FUNCTION "GESTIONE_ES" : VOID
TITLE =
{ S7_language := '9(1) Inglese (Stati Uniti)  11.01.2022  09:45:15' }
VERSION : 0.1


VAR_TEMP
  RETVAL : INT ;
  SetPointCamera_1 : REAL ;	//43FLA02 (camera riscaldo 1)
  SetPointCamera_2 : REAL ;	//44FLA02 (camera riscaldo 2)
  SetPointCamera_3 : REAL ;	//51FLA02 (camera riscaldo 3)
  SetPointCamera_4 : REAL ;	//52FLA02 (camera riscaldo 4)
  SetPointForno : REAL ;	//Forno
END_VAR
BEGIN
NETWORK
TITLE =**************************************

NETWORK
TITLE =Abilita Gestione Risparmio Energetico
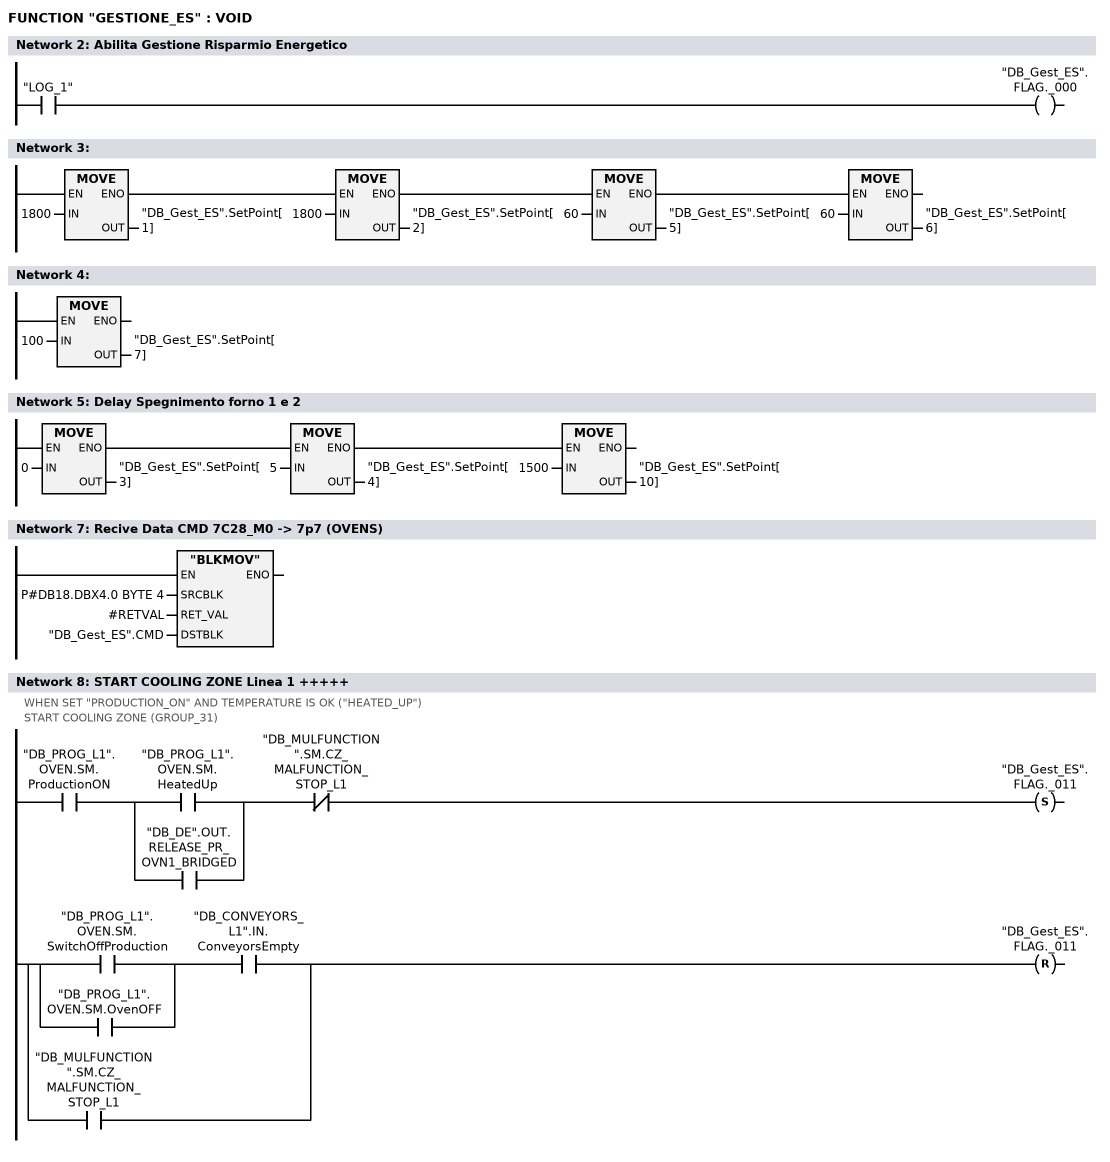
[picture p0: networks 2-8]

      U     "LOG_1";
      =     "DB_Gest_ES".FLAG._000;
NETWORK
TITLE =

      U(    ;
      U(    ;
      U(    ;
      L     1800;
      T     "DB_Gest_ES".SetPoint[1];
      SET   ;
      SAVE  ;
      CLR   ;
      U     BIE;
      )     ;
      SPBNB _001;
      L     1800;
      T     "DB_Gest_ES".SetPoint[2];
      SET   ;
      SAVE  ;
      CLR   ;
_001: U     BIE;
      )     ;
      SPBNB _002;
      L     60;
      T     "DB_Gest_ES".SetPoint[5];
      SET   ;
      SAVE  ;
      CLR   ;
_002: U     BIE;
      )     ;
      SPBNB _003;
      L     60;
      T     "DB_Gest_ES".SetPoint[6];
_003: NOP   0;
NETWORK
TITLE =

      L     100;
      T     "DB_Gest_ES".SetPoint[7];
      NOP   0;
NETWORK
TITLE =Delay Spegnimento forno 1 e 2

      U(    ;
      U(    ;
      L     0;
      T     "DB_Gest_ES".SetPoint[3];
      SET   ;
      SAVE  ;
      CLR   ;
      U     BIE;
      )     ;
      SPBNB _004;
      L     5;
      T     "DB_Gest_ES".SetPoint[4];
      SET   ;
      SAVE  ;
      CLR   ;
_004: U     BIE;
      )     ;
      SPBNB _005;
      L     1500;
      T     "DB_Gest_ES".SetPoint[10];
_005: NOP   0;
NETWORK
TITLE =**************************************

NETWORK
TITLE =Recive Data CMD 7C28_M0 -> 7p7 (OVENS)

      CALL "BLKMOV" (
           SRCBLK                   := P#DB18.DBX4.0 BYTE 4,
           RET_VAL                  := #RETVAL,
           DSTBLK                   := "DB_Gest_ES".CMD);
      NOP   0;
NETWORK
TITLE =START COOLING ZONE Linea 1 +++++
//WHEN SET "PRODUCTION_ON" AND TEMPERATURE IS OK ("HEATED_UP")
//START COOLING ZONE (GROUP_31)
      U     "DB_PROG_L1".OVEN.SM.ProductionON;
      U(    ;
      O     "DB_PROG_L1".OVEN.SM.HeatedUp;
      O     "DB_DE".OUT.RELEASE_PR_OVN1_BRIDGED;
      )     ;
      UN    "DB_MULFUNCTION".SM.CZ_MALFUNCTION_STOP_L1;
      S     "DB_Gest_ES".FLAG._011;
      U(    ;
      U(    ;
      O     "DB_PROG_L1".OVEN.SM.SwitchOffProduction;
      O     "DB_PROG_L1".OVEN.SM.OvenOFF;
      )     ;
      U     "DB_CONVEYORS_L1".IN.ConveyorsEmpty;
      O     "DB_MULFUNCTION".SM.CZ_MALFUNCTION_STOP_L1;
      )     ;
      R     "DB_Gest_ES".FLAG._011;
      NOP   0;
NETWORK
TITLE =Stop Raffreddamento Linea 1
//DB8.DBD38
      U     "DB_Gest_ES".FLAG._011;
      U     "DB_Gest_ES".FLAG._000;
      =     L     22.0;
      U     L     22.0;
      U(    ;
      U     "DB_Gest_ES".CMD.StopVentilazione_Zona1;
      UN    "DB_Gest_ES".FLAG._013;
      O     ;
      U     "DB_Gest_ES".Tmr.EN_Delay_01;
      UN    "DB_Gest_ES".Tmr.DN_Delay_01;
      )     ;
      S     "DB_Gest_ES".FLAG._001;
      U     L     22.0;
      UN    "DB_Gest_ES".CMD.StopVentilazione_Zona1;
      UN    "DB_Gest_ES".FLAG._013;
      S     "DB_Gest_ES".FLAG._013;
      U(    ;
      U     L     22.0;
      U     "DB_Gest_ES".CMD.VentilazioneRid_Zona1;
      =     "DB_Gest_ES".Tmr.EN_Delay_05;
      U     "DB_Gest_ES".Tmr.EN_Delay_05;
      )     ;
      U     "DB_Gest_ES".Tmr.DN_Delay_05;
      =     "DB_Gest_ES".FLAG._021;
NETWORK
TITLE =AUX Start Raff. Linea 1
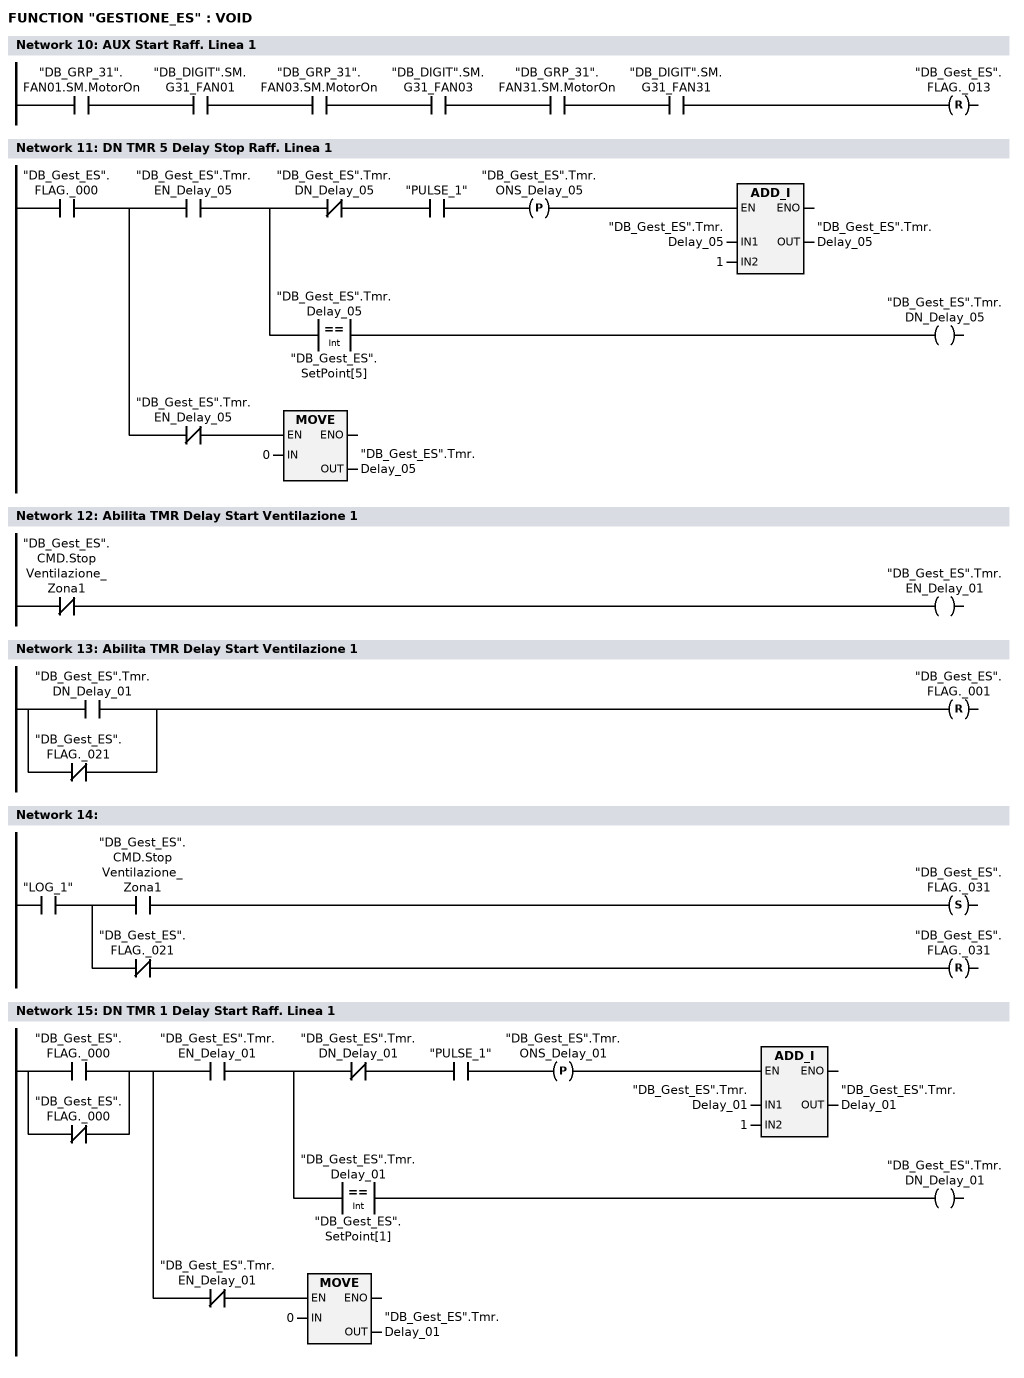
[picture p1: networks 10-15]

      U     "DB_GRP_31".FAN01.SM.MotorOn;
      U     "DB_DIGIT".SM.G31_FAN01;
      U     "DB_GRP_31".FAN03.SM.MotorOn;
      U     "DB_DIGIT".SM.G31_FAN03;
      U     "DB_GRP_31".FAN31.SM.MotorOn;
      U     "DB_DIGIT".SM.G31_FAN31;
      R     "DB_Gest_ES".FLAG._013;
NETWORK
TITLE =DN TMR 5 Delay Stop Raff. Linea 1

      U     "DB_Gest_ES".FLAG._000;
      =     L     22.0;
      U     L     22.0;
      U     "DB_Gest_ES".Tmr.EN_Delay_05;
      =     L     22.1;
      U     L     22.1;
      UN    "DB_Gest_ES".Tmr.DN_Delay_05;
      U     "PULSE_1";
      FP    "DB_Gest_ES".Tmr.ONS_Delay_05;
      SPBNB _006;
      L     "DB_Gest_ES".Tmr.Delay_05;
      L     1;
      +I    ;
      T     "DB_Gest_ES".Tmr.Delay_05;
_006: NOP   0;
      U     L     22.1;
      U(    ;
      L     "DB_Gest_ES".Tmr.Delay_05;
      L     "DB_Gest_ES".SetPoint[5];
      ==I   ;
      )     ;
      =     "DB_Gest_ES".Tmr.DN_Delay_05;
      U     L     22.0;
      UN    "DB_Gest_ES".Tmr.EN_Delay_05;
      SPBNB _007;
      L     0;
      T     "DB_Gest_ES".Tmr.Delay_05;
_007: NOP   0;
NETWORK
TITLE =Abilita TMR Delay Start Ventilazione 1

      UN    "DB_Gest_ES".CMD.StopVentilazione_Zona1;
      =     "DB_Gest_ES".Tmr.EN_Delay_01;
NETWORK
TITLE =Abilita TMR Delay Start Ventilazione 1

      O     "DB_Gest_ES".Tmr.DN_Delay_01;
      ON    "DB_Gest_ES".FLAG._021;
      R     "DB_Gest_ES".FLAG._001;
NETWORK
TITLE =

      U     "LOG_1";
      =     L     22.0;
      U     L     22.0;
      U     "DB_Gest_ES".CMD.StopVentilazione_Zona1;
      S     "DB_Gest_ES".FLAG._031;
      U     L     22.0;
      UN    "DB_Gest_ES".FLAG._021;
      R     "DB_Gest_ES".FLAG._031;
NETWORK
TITLE =DN TMR 1 Delay Start Raff. Linea 1

      O     "DB_Gest_ES".FLAG._000;
      ON    "DB_Gest_ES".FLAG._000;
      =     L     22.0;
      U     L     22.0;
      U     "DB_Gest_ES".Tmr.EN_Delay_01;
      =     L     22.1;
      U     L     22.1;
      UN    "DB_Gest_ES".Tmr.DN_Delay_01;
      U     "PULSE_1";
      FP    "DB_Gest_ES".Tmr.ONS_Delay_01;
      SPBNB _008;
      L     "DB_Gest_ES".Tmr.Delay_01;
      L     1;
      +I    ;
      T     "DB_Gest_ES".Tmr.Delay_01;
_008: NOP   0;
      U     L     22.1;
      U(    ;
      L     "DB_Gest_ES".Tmr.Delay_01;
      L     "DB_Gest_ES".SetPoint[1];
      ==I   ;
      )     ;
      =     "DB_Gest_ES".Tmr.DN_Delay_01;
      U     L     22.0;
      UN    "DB_Gest_ES".Tmr.EN_Delay_01;
      SPBNB _009;
      L     0;
      T     "DB_Gest_ES".Tmr.Delay_01;
_009: NOP   0;
NETWORK
TITLE =Stop Riscaldamento Linea 1

      U     "LOG_0";
      =     L     22.0;
      U(    ;
      U     L     22.0;
      U     "DB_Gest_ES".FLAG._000;
      U     "DB_CalendarioF1".CMD_OFF;
      U     "DB_CalendarioF1".Auto;
      UN    "DB_PROG_L1".OVEN.SM.SwitchOffProduction;
      U     "DB_Gest_ES".CMD.Stop_Riscarldo_Forno1;
      U     "DB_Gest_ES".CMD.AssenzaScoccheCabina;
      =     "DB_Gest_ES".Tmr.EN_Delay_03;
      U     "DB_Gest_ES".Tmr.EN_Delay_03;
      )     ;
      U     "DB_Gest_ES".Tmr.DN_Delay_03;
      S     "DB_Gest_ES".FLAG._003;
      R     "DB_CalendarioF1".CMD_OFF;
      U     L     22.0;
      U(    ;
      O     "DB_PROG_L1".OVEN.SM.SwitchOffProduction;
      O     "DB_PROG_L1".OVEN.SM.OvenOFF;
      O     "DB_PROG_L1".OVEN.CTRL.PreHeatingOn;
      O     "DB_PROG_L1".OVEN.CTRL.ProductionOn;
      )     ;
      R     "DB_Gest_ES".FLAG._003;
NETWORK
TITLE =
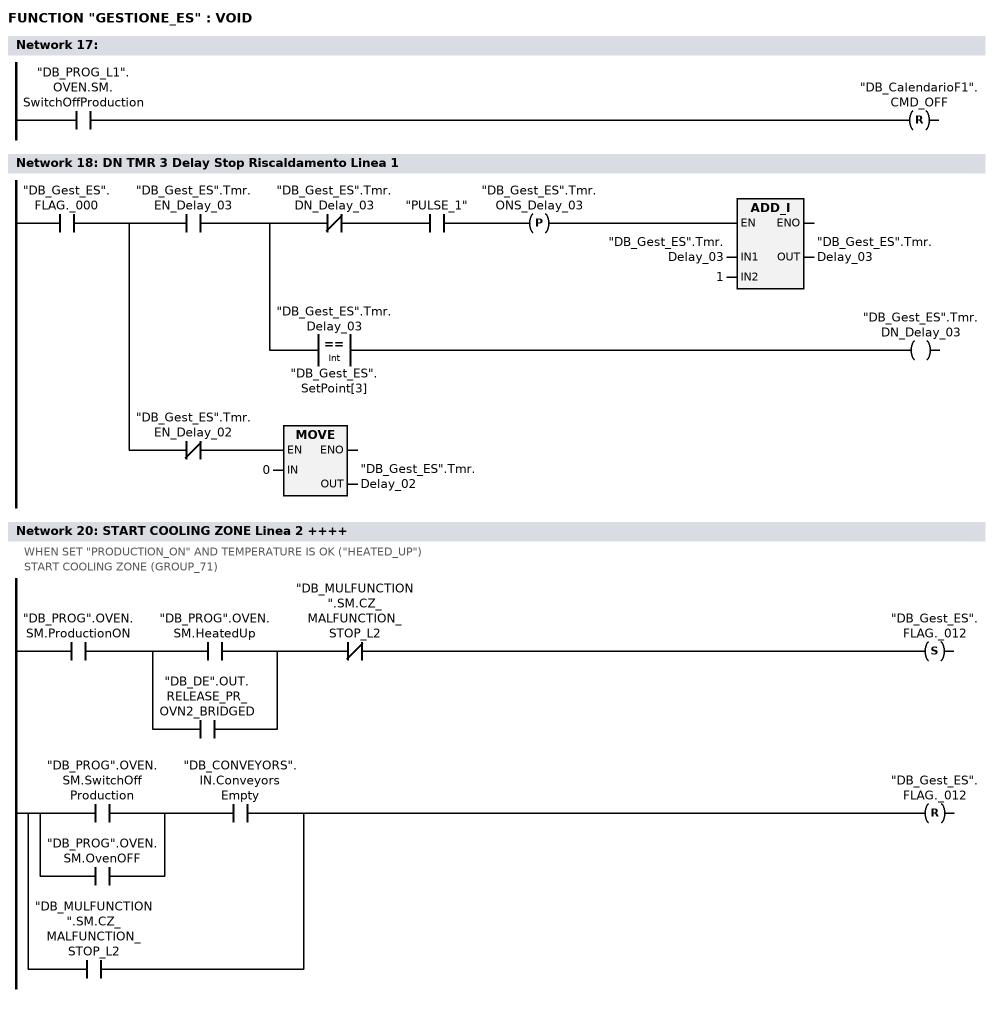
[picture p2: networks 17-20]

      U     "DB_PROG_L1".OVEN.SM.SwitchOffProduction;
      R     "DB_CalendarioF1".CMD_OFF;
NETWORK
TITLE =DN TMR 3 Delay Stop Riscaldamento Linea 1

      U     "DB_Gest_ES".FLAG._000;
      =     L     22.0;
      U     L     22.0;
      U     "DB_Gest_ES".Tmr.EN_Delay_03;
      =     L     22.1;
      U     L     22.1;
      UN    "DB_Gest_ES".Tmr.DN_Delay_03;
      U     "PULSE_1";
      FP    "DB_Gest_ES".Tmr.ONS_Delay_03;
      SPBNB _00a;
      L     "DB_Gest_ES".Tmr.Delay_03;
      L     1;
      +I    ;
      T     "DB_Gest_ES".Tmr.Delay_03;
_00a: NOP   0;
      U     L     22.1;
      U(    ;
      L     "DB_Gest_ES".Tmr.Delay_03;
      L     "DB_Gest_ES".SetPoint[3];
      ==I   ;
      )     ;
      =     "DB_Gest_ES".Tmr.DN_Delay_03;
      U     L     22.0;
      UN    "DB_Gest_ES".Tmr.EN_Delay_02;
      SPBNB _00b;
      L     0;
      T     "DB_Gest_ES".Tmr.Delay_02;
_00b: NOP   0;
NETWORK
TITLE =**************************************

NETWORK
TITLE =START COOLING ZONE Linea 2 ++++
//WHEN SET "PRODUCTION_ON" AND TEMPERATURE IS OK ("HEATED_UP")
//START COOLING ZONE (GROUP_71)
      U     "DB_PROG".OVEN.SM.ProductionON;
      U(    ;
      O     "DB_PROG".OVEN.SM.HeatedUp;
      O     "DB_DE".OUT.RELEASE_PR_OVN2_BRIDGED;
      )     ;
      UN    "DB_MULFUNCTION".SM.CZ_MALFUNCTION_STOP_L2;
      S     "DB_Gest_ES".FLAG._012;
      U(    ;
      U(    ;
      O     "DB_PROG".OVEN.SM.SwitchOffProduction;
      O     "DB_PROG".OVEN.SM.OvenOFF;
      )     ;
      U     "DB_CONVEYORS".IN.ConveyorsEmpty;
      O     "DB_MULFUNCTION".SM.CZ_MALFUNCTION_STOP_L2;
      )     ;
      R     "DB_Gest_ES".FLAG._012;
      NOP   0;
NETWORK
TITLE =Stop Raffreddamento Linea 2
//DB8.DBD38
      U     "DB_Gest_ES".FLAG._012;
      U     "DB_Gest_ES".FLAG._000;
      U     "LOG_0";
      =     L     22.0;
      U     L     22.0;
      U(    ;
      U     "DB_Gest_ES".CMD.StopVentilazione_Zona2;
      UN    "DB_Gest_ES".FLAG._014;
      O     ;
      U     "DB_Gest_ES".Tmr.EN_Delay_02;
      UN    "DB_Gest_ES".Tmr.DN_Delay_02;
      )     ;
      S     "DB_Gest_ES".FLAG._002;
      U     L     22.0;
      UN    "DB_Gest_ES".CMD.StopVentilazione_Zona2;
      UN    "DB_Gest_ES".FLAG._014;
      S     "DB_Gest_ES".FLAG._014;
      U(    ;
      U     L     22.0;
      U     "DB_Gest_ES".CMD.VentilazioneRid_Zona2;
      =     "DB_Gest_ES".Tmr.EN_Delay_06;
      U     "DB_Gest_ES".Tmr.EN_Delay_06;
      )     ;
      U     "DB_Gest_ES".Tmr.DN_Delay_06;
      =     "DB_Gest_ES".FLAG._022;
NETWORK
TITLE =AUX Start Raff. Linea 2
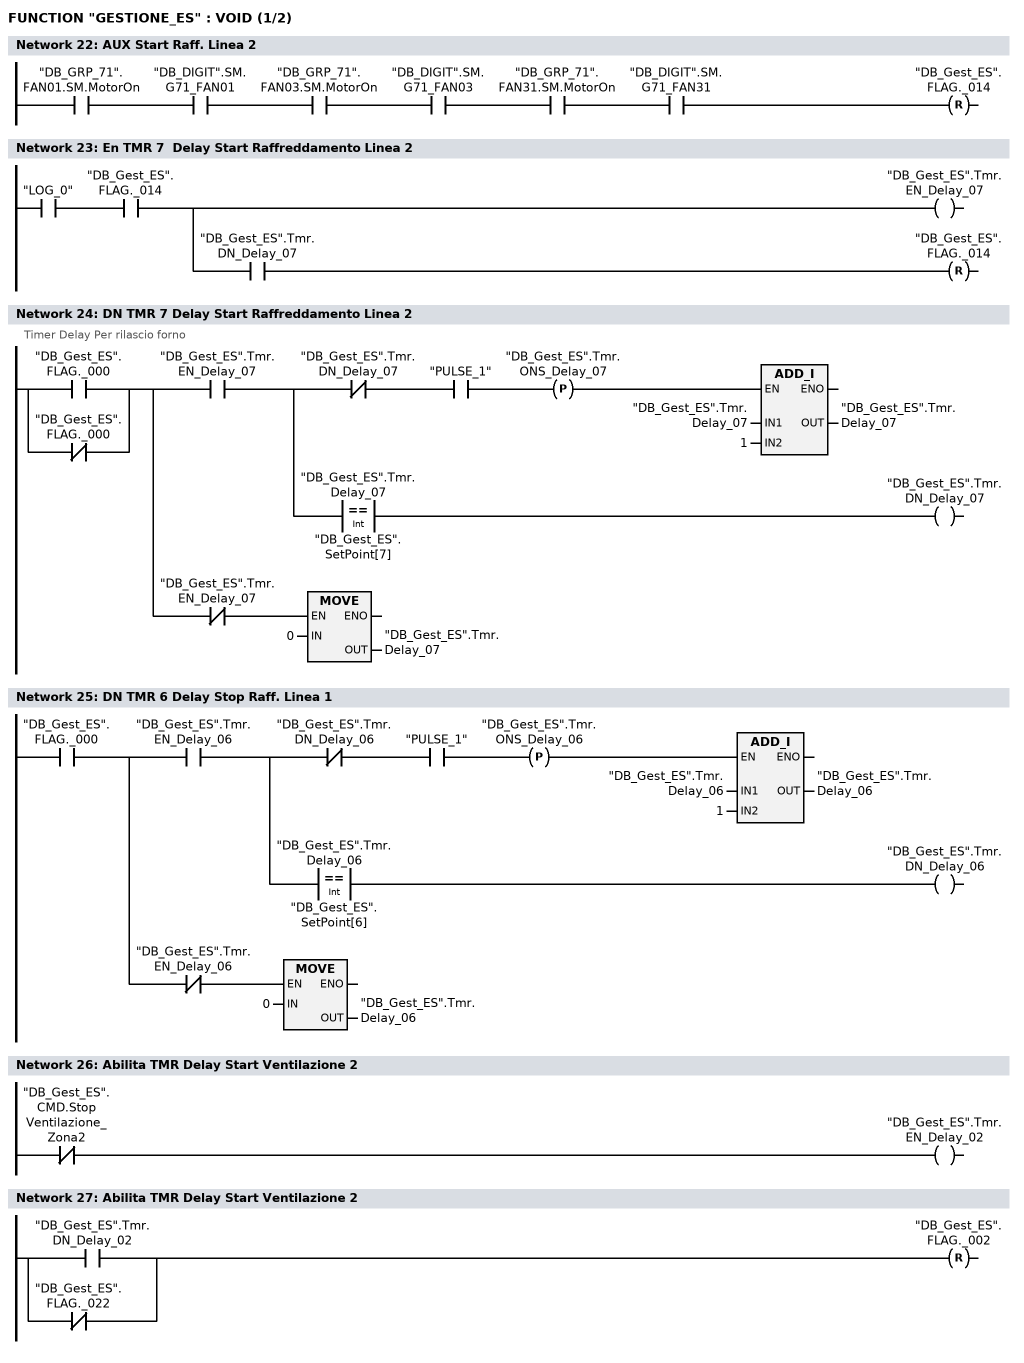
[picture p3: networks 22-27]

      U     "DB_GRP_71".FAN01.SM.MotorOn;
      U     "DB_DIGIT".SM.G71_FAN01;
      U     "DB_GRP_71".FAN03.SM.MotorOn;
      U     "DB_DIGIT".SM.G71_FAN03;
      U     "DB_GRP_71".FAN31.SM.MotorOn;
      U     "DB_DIGIT".SM.G71_FAN31;
      R     "DB_Gest_ES".FLAG._014;
NETWORK
TITLE =En TMR 7  Delay Start Raffreddamento Linea 2

      U     "LOG_0";
      U     "DB_Gest_ES".FLAG._014;
      =     L     22.0;
      U     L     22.0;
      BLD   102;
      =     "DB_Gest_ES".Tmr.EN_Delay_07;
      U     L     22.0;
      U     "DB_Gest_ES".Tmr.DN_Delay_07;
      R     "DB_Gest_ES".FLAG._014;
NETWORK
TITLE =DN TMR 7 Delay Start Raffreddamento Linea 2
//Timer Delay Per rilascio forno
      O     "DB_Gest_ES".FLAG._000;
      ON    "DB_Gest_ES".FLAG._000;
      =     L     22.0;
      U     L     22.0;
      U     "DB_Gest_ES".Tmr.EN_Delay_07;
      =     L     22.1;
      U     L     22.1;
      UN    "DB_Gest_ES".Tmr.DN_Delay_07;
      U     "PULSE_1";
      FP    "DB_Gest_ES".Tmr.ONS_Delay_07;
      SPBNB _00c;
      L     "DB_Gest_ES".Tmr.Delay_07;
      L     1;
      +I    ;
      T     "DB_Gest_ES".Tmr.Delay_07;
_00c: NOP   0;
      U     L     22.1;
      U(    ;
      L     "DB_Gest_ES".Tmr.Delay_07;
      L     "DB_Gest_ES".SetPoint[7];
      ==I   ;
      )     ;
      =     "DB_Gest_ES".Tmr.DN_Delay_07;
      U     L     22.0;
      UN    "DB_Gest_ES".Tmr.EN_Delay_07;
      SPBNB _00d;
      L     0;
      T     "DB_Gest_ES".Tmr.Delay_07;
_00d: NOP   0;
NETWORK
TITLE =DN TMR 6 Delay Stop Raff. Linea 1

      U     "DB_Gest_ES".FLAG._000;
      =     L     22.0;
      U     L     22.0;
      U     "DB_Gest_ES".Tmr.EN_Delay_06;
      =     L     22.1;
      U     L     22.1;
      UN    "DB_Gest_ES".Tmr.DN_Delay_06;
      U     "PULSE_1";
      FP    "DB_Gest_ES".Tmr.ONS_Delay_06;
      SPBNB _00e;
      L     "DB_Gest_ES".Tmr.Delay_06;
      L     1;
      +I    ;
      T     "DB_Gest_ES".Tmr.Delay_06;
_00e: NOP   0;
      U     L     22.1;
      U(    ;
      L     "DB_Gest_ES".Tmr.Delay_06;
      L     "DB_Gest_ES".SetPoint[6];
      ==I   ;
      )     ;
      =     "DB_Gest_ES".Tmr.DN_Delay_06;
      U     L     22.0;
      UN    "DB_Gest_ES".Tmr.EN_Delay_06;
      SPBNB _00f;
      L     0;
      T     "DB_Gest_ES".Tmr.Delay_06;
_00f: NOP   0;
NETWORK
TITLE =Abilita TMR Delay Start Ventilazione 2

      UN    "DB_Gest_ES".CMD.StopVentilazione_Zona2;
      =     "DB_Gest_ES".Tmr.EN_Delay_02;
NETWORK
TITLE =Abilita TMR Delay Start Ventilazione 2

      O     "DB_Gest_ES".Tmr.DN_Delay_02;
      ON    "DB_Gest_ES".FLAG._022;
      R     "DB_Gest_ES".FLAG._002;
NETWORK
TITLE =DN TMR 2 Delay Stop Riscaldamento Linea 2
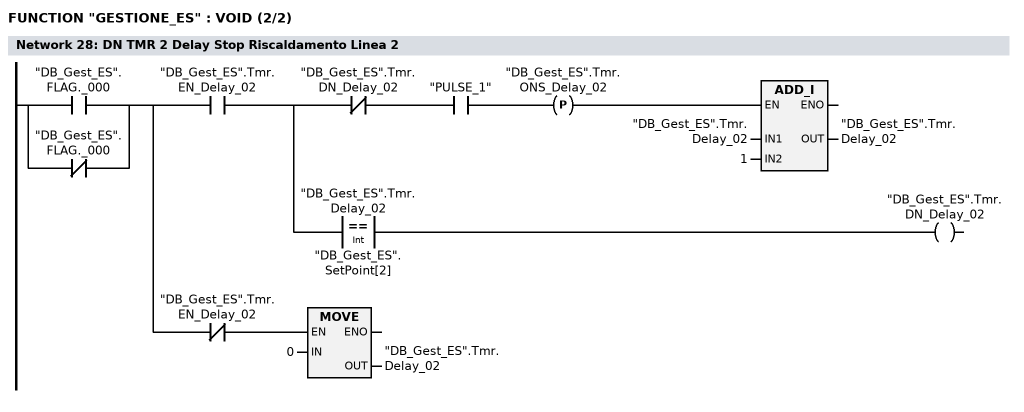
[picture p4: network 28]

      O     "DB_Gest_ES".FLAG._000;
      ON    "DB_Gest_ES".FLAG._000;
      =     L     22.0;
      U     L     22.0;
      U     "DB_Gest_ES".Tmr.EN_Delay_02;
      =     L     22.1;
      U     L     22.1;
      UN    "DB_Gest_ES".Tmr.DN_Delay_02;
      U     "PULSE_1";
      FP    "DB_Gest_ES".Tmr.ONS_Delay_02;
      SPBNB _010;
      L     "DB_Gest_ES".Tmr.Delay_02;
      L     1;
      +I    ;
      T     "DB_Gest_ES".Tmr.Delay_02;
_010: NOP   0;
      U     L     22.1;
      U(    ;
      L     "DB_Gest_ES".Tmr.Delay_02;
      L     "DB_Gest_ES".SetPoint[2];
      ==I   ;
      )     ;
      =     "DB_Gest_ES".Tmr.DN_Delay_02;
      U     L     22.0;
      UN    "DB_Gest_ES".Tmr.EN_Delay_02;
      SPBNB _011;
      L     0;
      T     "DB_Gest_ES".Tmr.Delay_02;
_011: NOP   0;
NETWORK
TITLE =Stop Riscaldamento Linea 2

      U     "LOG_1";
      =     L     22.0;
      U(    ;
      U     L     22.0;
      U     "DB_Gest_ES".FLAG._000;
      U     "DB_CalendarioF2".CMD_OFF;
      U     "DB_CalendarioF2".Auto;
      UN    "DB_PROG".OVEN.SM.SwitchOffProduction;
      U     "DB_Gest_ES".CMD.AssenzaScoccheCabina;
      =     "DB_Gest_ES".Tmr.EN_Delay_04;
      U     "DB_Gest_ES".Tmr.EN_Delay_04;
      )     ;
      U     "DB_Gest_ES".CMD.Stop_Riscarldo_Forno2;
      U     "DB_Gest_ES".Tmr.DN_Delay_04;
      U     "DB_Gest_ES".Tmr.DN_Delay_10;
      S     "DB_Gest_ES".FLAG._004;
      S     "DB_Gest_ES".FLAG._005;
      R     "DB_CalendarioF2".CMD_OFF;
      R     "DB_Gest_ES".FLAG._050;
      U     L     22.0;
      U(    ;
      U     "DB_PROG".OVEN.SM.SwitchOffProduction;
      UN    "DB_PROG".OVEN.SM.ProductionON;
      O     "DB_PROG".OVEN.SM.OvenOFF;
      O     "DB_PROG".OVEN.CTRL.PreHeatingOn;
      O     "DB_PROG".OVEN.CTRL.ProductionOn;
      )     ;
      R     "DB_Gest_ES".FLAG._004;
NETWORK
TITLE =RESET COMANDO OFF
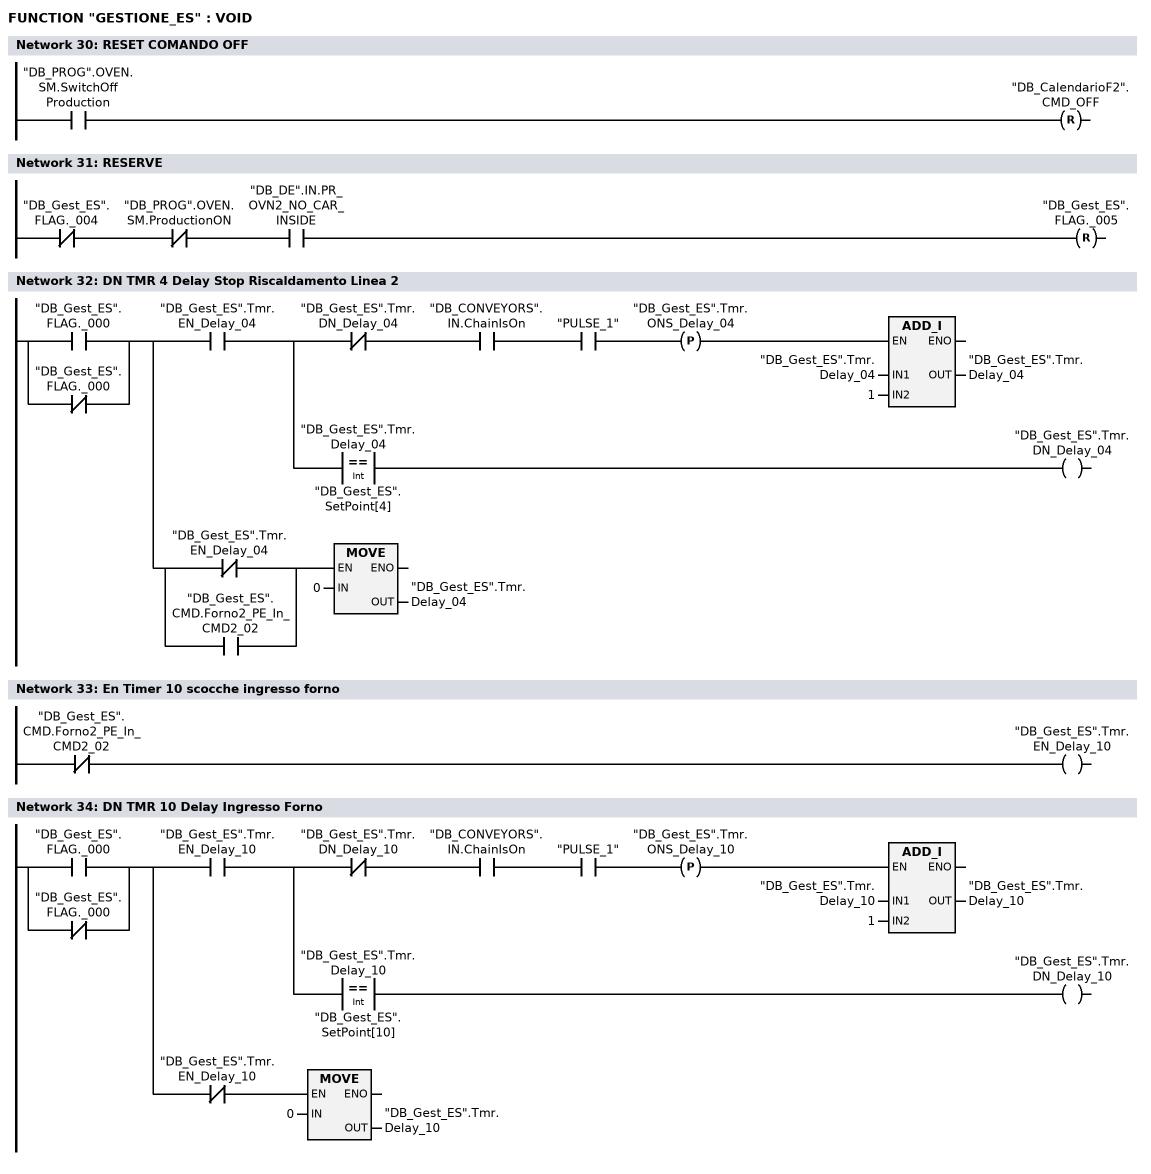
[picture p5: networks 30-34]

      U     "DB_PROG".OVEN.SM.SwitchOffProduction;
      R     "DB_CalendarioF2".CMD_OFF;
NETWORK
TITLE =RESERVE

      UN    "DB_Gest_ES".FLAG._004;
      UN    "DB_PROG".OVEN.SM.ProductionON;
      U     "DB_DE".IN.PR_OVN2_NO_CAR_INSIDE;
      R     "DB_Gest_ES".FLAG._005;
NETWORK
TITLE =DN TMR 4 Delay Stop Riscaldamento Linea 2

      O     "DB_Gest_ES".FLAG._000;
      ON    "DB_Gest_ES".FLAG._000;
      =     L     22.0;
      U     L     22.0;
      U     "DB_Gest_ES".Tmr.EN_Delay_04;
      =     L     22.1;
      U     L     22.1;
      UN    "DB_Gest_ES".Tmr.DN_Delay_04;
      U     "DB_CONVEYORS".IN.ChainIsOn;
      U     "PULSE_1";
      FP    "DB_Gest_ES".Tmr.ONS_Delay_04;
      SPBNB _012;
      L     "DB_Gest_ES".Tmr.Delay_04;
      L     1;
      +I    ;
      T     "DB_Gest_ES".Tmr.Delay_04;
_012: NOP   0;
      U     L     22.1;
      U(    ;
      L     "DB_Gest_ES".Tmr.Delay_04;
      L     "DB_Gest_ES".SetPoint[4];
      ==I   ;
      )     ;
      =     "DB_Gest_ES".Tmr.DN_Delay_04;
      U     L     22.0;
      U(    ;
      ON    "DB_Gest_ES".Tmr.EN_Delay_04;
      O     "DB_Gest_ES".CMD.Forno2_PE_In_CMD2_02;
      )     ;
      SPBNB _013;
      L     0;
      T     "DB_Gest_ES".Tmr.Delay_04;
_013: NOP   0;
NETWORK
TITLE =En Timer 10 scocche ingresso forno

      UN    "DB_Gest_ES".CMD.Forno2_PE_In_CMD2_02;
      =     "DB_Gest_ES".Tmr.EN_Delay_10;
NETWORK
TITLE =DN TMR 10 Delay Ingresso Forno

      O     "DB_Gest_ES".FLAG._000;
      ON    "DB_Gest_ES".FLAG._000;
      =     L     22.0;
      U     L     22.0;
      U     "DB_Gest_ES".Tmr.EN_Delay_10;
      =     L     22.1;
      U     L     22.1;
      UN    "DB_Gest_ES".Tmr.DN_Delay_10;
      U     "DB_CONVEYORS".IN.ChainIsOn;
      U     "PULSE_1";
      FP    "DB_Gest_ES".Tmr.ONS_Delay_10;
      SPBNB _014;
      L     "DB_Gest_ES".Tmr.Delay_10;
      L     1;
      +I    ;
      T     "DB_Gest_ES".Tmr.Delay_10;
_014: NOP   0;
      U     L     22.1;
      U(    ;
      L     "DB_Gest_ES".Tmr.Delay_10;
      L     "DB_Gest_ES".SetPoint[10];
      ==I   ;
      )     ;
      =     "DB_Gest_ES".Tmr.DN_Delay_10;
      U     L     22.0;
      UN    "DB_Gest_ES".Tmr.EN_Delay_10;
      SPBNB _015;
      L     0;
      T     "DB_Gest_ES".Tmr.Delay_10;
_015: NOP   0;
NETWORK
TITLE =**************************************

NETWORK
TITLE =######################################

NETWORK
TITLE =Send Data CMD 7P7 -> 7C28_M0

NETWORK
TITLE =######################################

NETWORK
TITLE =#CALENDARIO FORNO 1

NETWORK
TITLE =Set
//Anno
      L     DB3100.DBB    8;
      T     "DB_CalendarioF1".PLC.Year;
//Mese
      L     DB3100.DBB    9;
      T     "DB_CalendarioF1".PLC.Mon;
//Giorno
      L     DB3100.DBB   10;
      T     "DB_CalendarioF1".PLC.Day;


//Ore
      L     DB3100.DBB   11;
      BTI   ;
      T     "DB_CalendarioF1".PLC.Hour;
//Minuti
      L     DB3100.DBB   12;
      BTI   ;
      T     "DB_CalendarioF1".PLC.Min;



NETWORK
TITLE =Calcolo del giorno della settimana

      L     DB3100.DBB   15;
      UW    W#16#F;
      T     "DB_CalendarioF1".PLC.WeekDay;
NETWORK
TITLE =Richiamo FC Gestione calendario
//P#DB101.DBX 50.0 BYTE 4
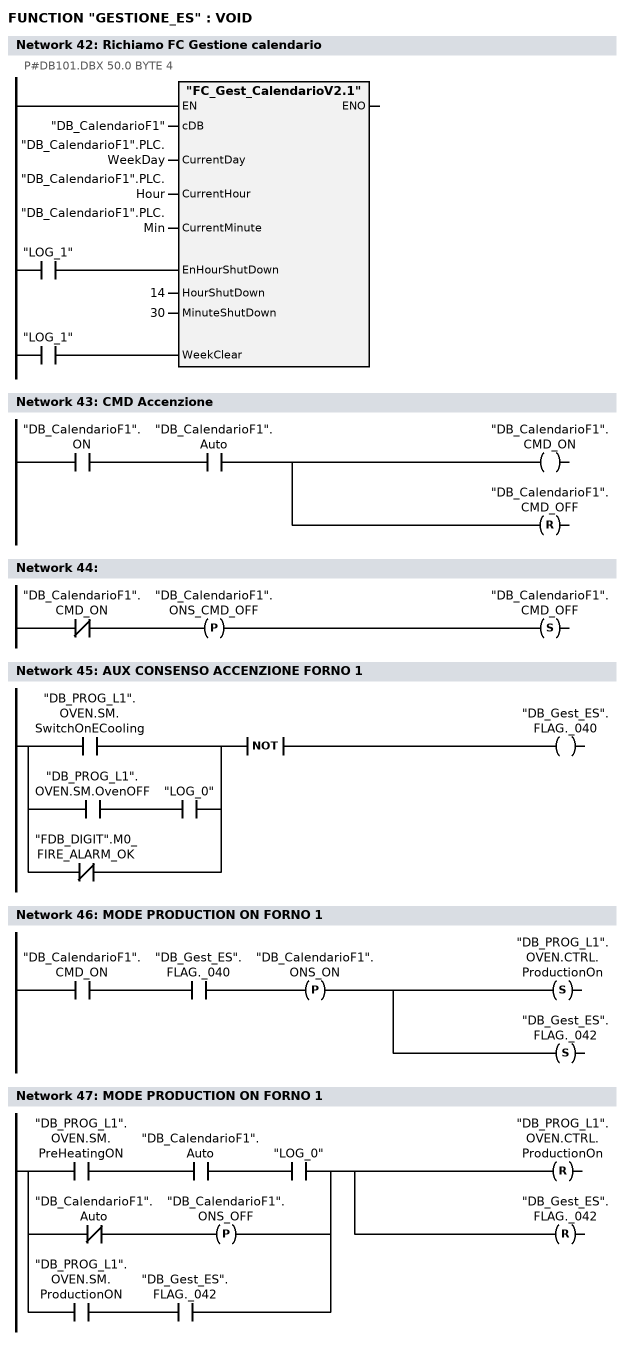
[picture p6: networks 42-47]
      U     "LOG_1";
      =     L     22.0;
      BLD   103;
      U     "LOG_1";
      =     L     22.1;
      BLD   103;
      CALL "FC_Gest_CalendarioV2.1" (
           cDB                      := "DB_CalendarioF1",
           CurrentDay               := "DB_CalendarioF1".PLC.WeekDay,
           CurrentHour              := "DB_CalendarioF1".PLC.Hour,
           CurrentMinute            := "DB_CalendarioF1".PLC.Min,
           EnHourShutDown           := L     22.0,
           HourShutDown             := 14,
           MinuteShutDown           := 30,
           WeekClear                := L     22.1);
      NOP   0;
NETWORK
TITLE =CMD Accenzione

      U     "DB_CalendarioF1".ON;
      U     "DB_CalendarioF1".Auto;
      =     "DB_CalendarioF1".CMD_ON;
      R     "DB_CalendarioF1".CMD_OFF;
NETWORK
TITLE =

      UN    "DB_CalendarioF1".CMD_ON;
      FP    "DB_CalendarioF1".ONS_CMD_OFF;
      S     "DB_CalendarioF1".CMD_OFF;
NETWORK
TITLE =AUX CONSENSO ACCENZIONE FORNO 1

      U(    ;
      O     "DB_PROG_L1".OVEN.SM.SwitchOnECooling;
      O     ;
      U     "DB_PROG_L1".OVEN.SM.OvenOFF;
      U     "LOG_0";
      ON    "FDB_DIGIT".M0_FIRE_ALARM_OK;
      )     ;
      NOT   ;
      =     "DB_Gest_ES".FLAG._040;
NETWORK
TITLE =MODE PRODUCTION ON FORNO 1

      U     "DB_CalendarioF1".CMD_ON;
      U     "DB_Gest_ES".FLAG._040;
      FP    "DB_CalendarioF1".ONS_ON;
      S     "DB_PROG_L1".OVEN.CTRL.ProductionOn;
      S     "DB_Gest_ES".FLAG._042;
NETWORK
TITLE =MODE PRODUCTION ON FORNO 1

      U     "DB_PROG_L1".OVEN.SM.PreHeatingON;
      U     "DB_CalendarioF1".Auto;
      U     "LOG_0";
      O(    ;
      UN    "DB_CalendarioF1".Auto;
      FP    "DB_CalendarioF1".ONS_OFF;
      )     ;
      O     ;
      U     "DB_PROG_L1".OVEN.SM.ProductionON;
      U     "DB_Gest_ES".FLAG._042;
      R     "DB_PROG_L1".OVEN.CTRL.ProductionOn;
      R     "DB_Gest_ES".FLAG._042;
NETWORK
TITLE =######################################

NETWORK
TITLE =#CALENDARIO FORNO 2

NETWORK
TITLE =Set
//Anno
      L     DB3100.DBB    8;
      T     "DB_CalendarioF2".PLC.Year;
//Mese
      L     DB3100.DBB    9;
      T     "DB_CalendarioF2".PLC.Mon;
//Giorno
      L     DB3100.DBB   10;
      T     "DB_CalendarioF2".PLC.Day;


//Ore
      L     DB3100.DBB   11;
      BTI   ;
      T     "DB_CalendarioF2".PLC.Hour;
//Minuti
      L     DB3100.DBB   12;
      BTI   ;
      T     "DB_CalendarioF2".PLC.Min;



NETWORK
TITLE =Calcolo del giorno della settimana

      L     DB3100.DBB   15;
      UW    W#16#F;
      T     "DB_CalendarioF2".PLC.WeekDay;
NETWORK
TITLE =Richiamo FC Gestione calendario
//P#DB101.DBX 50.0 BYTE 4
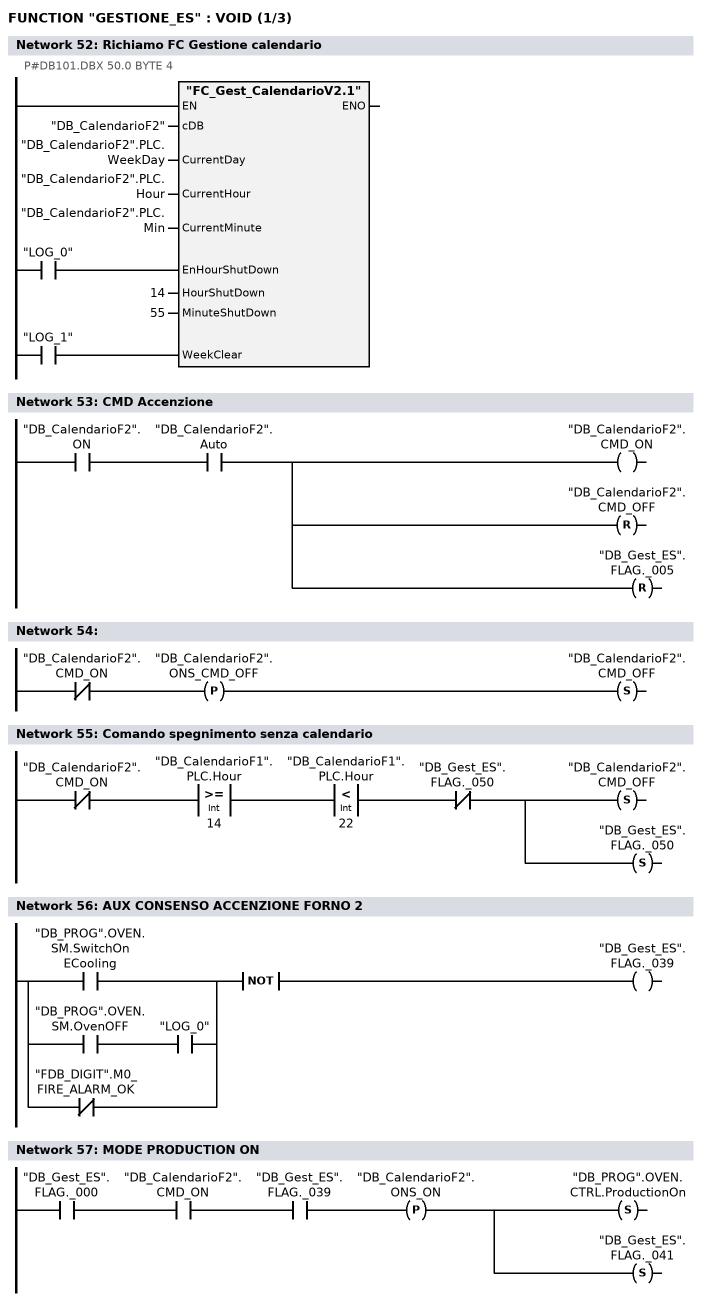
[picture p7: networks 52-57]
      U     "LOG_0";
      =     L     22.0;
      BLD   103;
      U     "LOG_1";
      =     L     22.1;
      BLD   103;
      CALL "FC_Gest_CalendarioV2.1" (
           cDB                      := "DB_CalendarioF2",
           CurrentDay               := "DB_CalendarioF2".PLC.WeekDay,
           CurrentHour              := "DB_CalendarioF2".PLC.Hour,
           CurrentMinute            := "DB_CalendarioF2".PLC.Min,
           EnHourShutDown           := L     22.0,
           HourShutDown             := 14,
           MinuteShutDown           := 55,
           WeekClear                := L     22.1);
      NOP   0;
NETWORK
TITLE =CMD Accenzione

      U     "DB_CalendarioF2".ON;
      U     "DB_CalendarioF2".Auto;
      =     "DB_CalendarioF2".CMD_ON;
      R     "DB_CalendarioF2".CMD_OFF;
      R     "DB_Gest_ES".FLAG._005;
NETWORK
TITLE =

      UN    "DB_CalendarioF2".CMD_ON;
      FP    "DB_CalendarioF2".ONS_CMD_OFF;
      S     "DB_CalendarioF2".CMD_OFF;
NETWORK
TITLE =Comando spegnimento senza calendario

      UN    "DB_CalendarioF2".CMD_ON;
      U(    ;
      L     "DB_CalendarioF1".PLC.Hour;
      L     14;
      >=I   ;
      )     ;
      U(    ;
      L     "DB_CalendarioF1".PLC.Hour;
      L     22;
      <I    ;
      )     ;
      UN    "DB_Gest_ES".FLAG._050;
      S     "DB_CalendarioF2".CMD_OFF;
      S     "DB_Gest_ES".FLAG._050;
NETWORK
TITLE =AUX CONSENSO ACCENZIONE FORNO 2

      U(    ;
      O     "DB_PROG".OVEN.SM.SwitchOnECooling;
      O     ;
      U     "DB_PROG".OVEN.SM.OvenOFF;
      U     "LOG_0";
      ON    "FDB_DIGIT".M0_FIRE_ALARM_OK;
      )     ;
      NOT   ;
      =     "DB_Gest_ES".FLAG._039;
NETWORK
TITLE =MODE PRODUCTION ON

      U     "DB_Gest_ES".FLAG._000;
      U     "DB_CalendarioF2".CMD_ON;
      U     "DB_Gest_ES".FLAG._039;
      FP    "DB_CalendarioF2".ONS_ON;
      S     "DB_PROG".OVEN.CTRL.ProductionOn;
      S     "DB_Gest_ES".FLAG._041;
NETWORK
TITLE =MODE PRODUCTION ON
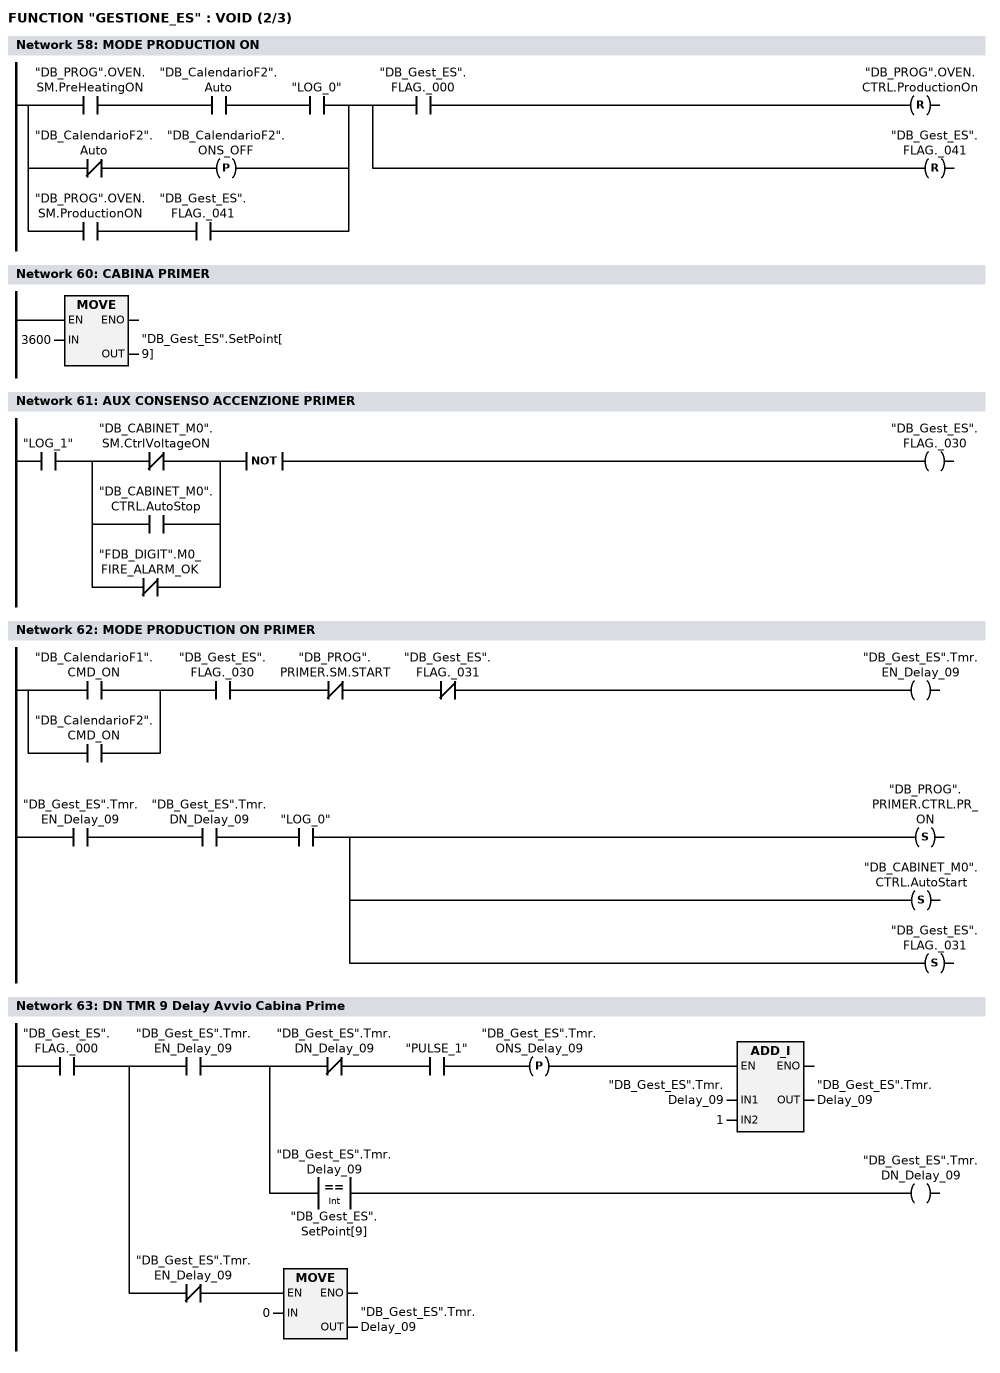
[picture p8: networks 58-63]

      U     "DB_PROG".OVEN.SM.PreHeatingON;
      U     "DB_CalendarioF2".Auto;
      U     "LOG_0";
      O(    ;
      UN    "DB_CalendarioF2".Auto;
      FP    "DB_CalendarioF2".ONS_OFF;
      )     ;
      O     ;
      U     "DB_PROG".OVEN.SM.ProductionON;
      U     "DB_Gest_ES".FLAG._041;
      =     L     22.0;
      U     L     22.0;
      U     "DB_Gest_ES".FLAG._000;
      R     "DB_PROG".OVEN.CTRL.ProductionOn;
      U     L     22.0;
      BLD   102;
      R     "DB_Gest_ES".FLAG._041;
NETWORK
TITLE =######################################

NETWORK
TITLE =CABINA PRIMER

      L     3600;
      T     "DB_Gest_ES".SetPoint[9];
      NOP   0;
NETWORK
TITLE =AUX CONSENSO ACCENZIONE PRIMER

      U     "LOG_1";
      U(    ;
      ON    "DB_CABINET_M0".SM.CtrlVoltageON;
      O     "DB_CABINET_M0".CTRL.AutoStop;
      ON    "FDB_DIGIT".M0_FIRE_ALARM_OK;
      )     ;
      NOT   ;
      =     "DB_Gest_ES".FLAG._030;
NETWORK
TITLE =MODE PRODUCTION ON PRIMER

      U(    ;
      O     "DB_CalendarioF1".CMD_ON;
      O     "DB_CalendarioF2".CMD_ON;
      )     ;
      U     "DB_Gest_ES".FLAG._030;
      UN    "DB_PROG".PRIMER.SM.START;
      UN    "DB_Gest_ES".FLAG._031;
      =     "DB_Gest_ES".Tmr.EN_Delay_09;
      U     "DB_Gest_ES".Tmr.EN_Delay_09;
      U     "DB_Gest_ES".Tmr.DN_Delay_09;
      U     "LOG_0";
      S     "DB_PROG".PRIMER.CTRL.PR_ON;
      S     "DB_CABINET_M0".CTRL.AutoStart;
      S     "DB_Gest_ES".FLAG._031;
NETWORK
TITLE =DN TMR 9 Delay Avvio Cabina Prime

      U     "DB_Gest_ES".FLAG._000;
      =     L     22.0;
      U     L     22.0;
      U     "DB_Gest_ES".Tmr.EN_Delay_09;
      =     L     22.1;
      U     L     22.1;
      UN    "DB_Gest_ES".Tmr.DN_Delay_09;
      U     "PULSE_1";
      FP    "DB_Gest_ES".Tmr.ONS_Delay_09;
      SPBNB _016;
      L     "DB_Gest_ES".Tmr.Delay_09;
      L     1;
      +I    ;
      T     "DB_Gest_ES".Tmr.Delay_09;
_016: NOP   0;
      U     L     22.1;
      U(    ;
      L     "DB_Gest_ES".Tmr.Delay_09;
      L     "DB_Gest_ES".SetPoint[9];
      ==I   ;
      )     ;
      =     "DB_Gest_ES".Tmr.DN_Delay_09;
      U     L     22.0;
      UN    "DB_Gest_ES".Tmr.EN_Delay_09;
      SPBNB _017;
      L     0;
      T     "DB_Gest_ES".Tmr.Delay_09;
_017: NOP   0;
NETWORK
TITLE =MODE PRODUCTION ON PRIMER
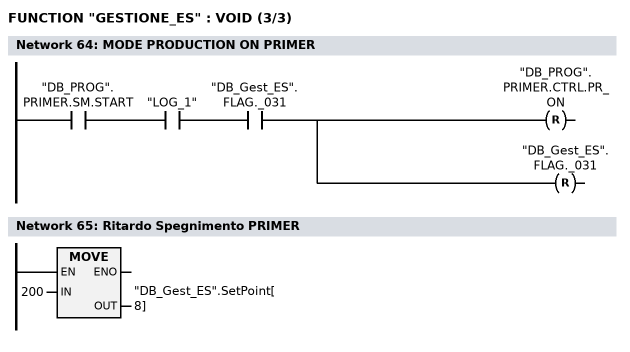
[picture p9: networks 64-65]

      U     "DB_PROG".PRIMER.SM.START;
      U     "LOG_1";
      U     "DB_Gest_ES".FLAG._031;
      R     "DB_PROG".PRIMER.CTRL.PR_ON;
      R     "DB_Gest_ES".FLAG._031;
NETWORK
TITLE =Ritardo Spegnimento PRIMER

      L     200;
      T     "DB_Gest_ES".SetPoint[8];
      NOP   0;
NETWORK
TITLE =Stop CABINA PRIMER

      U     "LOG_0";
      =     L     22.0;
      U(    ;
      U     L     22.0;
      U     "DB_Gest_ES".FLAG._000;
      U     "DB_PROG".PRIMER.SM.ON;
      UN    "DB_Gest_ES".FLAG._033;
      U     "DB_CalendarioF2".Auto;
      U     "DB_CalendarioF1".Auto;
      UN    "DB_CalendarioF1".CMD_ON;
      UN    "DB_CalendarioF2".CMD_ON;
      UN    "DB_PROG".OVEN.CTRL.ProductionOn;
      UN    "DB_PROG_L1".OVEN.CTRL.ProductionOn;
      U(    ;
      ON    "DB_PROG".OVEN.SM.ProductionON;
      O     "DB_PROG".OVEN.SM.ProductionON;
      )     ;
      U(    ;
      ON    "DB_PROG_L1".OVEN.SM.ProductionON;
      O     "DB_PROG_L1".OVEN.SM.ProductionON;
      )     ;
      U     "DB_Gest_ES".CMD.AssenzaScoccheCabina;
      =     "DB_Gest_ES".Tmr.EN_Delay_08;
      U     "DB_Gest_ES".Tmr.EN_Delay_08;
      )     ;
      U     "DB_Gest_ES".Tmr.DN_Delay_08;
      S     "DB_Gest_ES".FLAG._032;
      R     "DB_PROG".PRIMER.SM.ON;
      S     "DB_CABINET_M0".CTRL.AutoStop;
      S     "DB_PROG".PRIMER.SM.STOP;
      U     L     22.0;
      UN    "DB_PROG".PRIMER.SM.ON;
      U     "DB_Gest_ES".FLAG._032;
      R     "DB_Gest_ES".FLAG._032;
NETWORK
TITLE =Reset CMD Clean Room
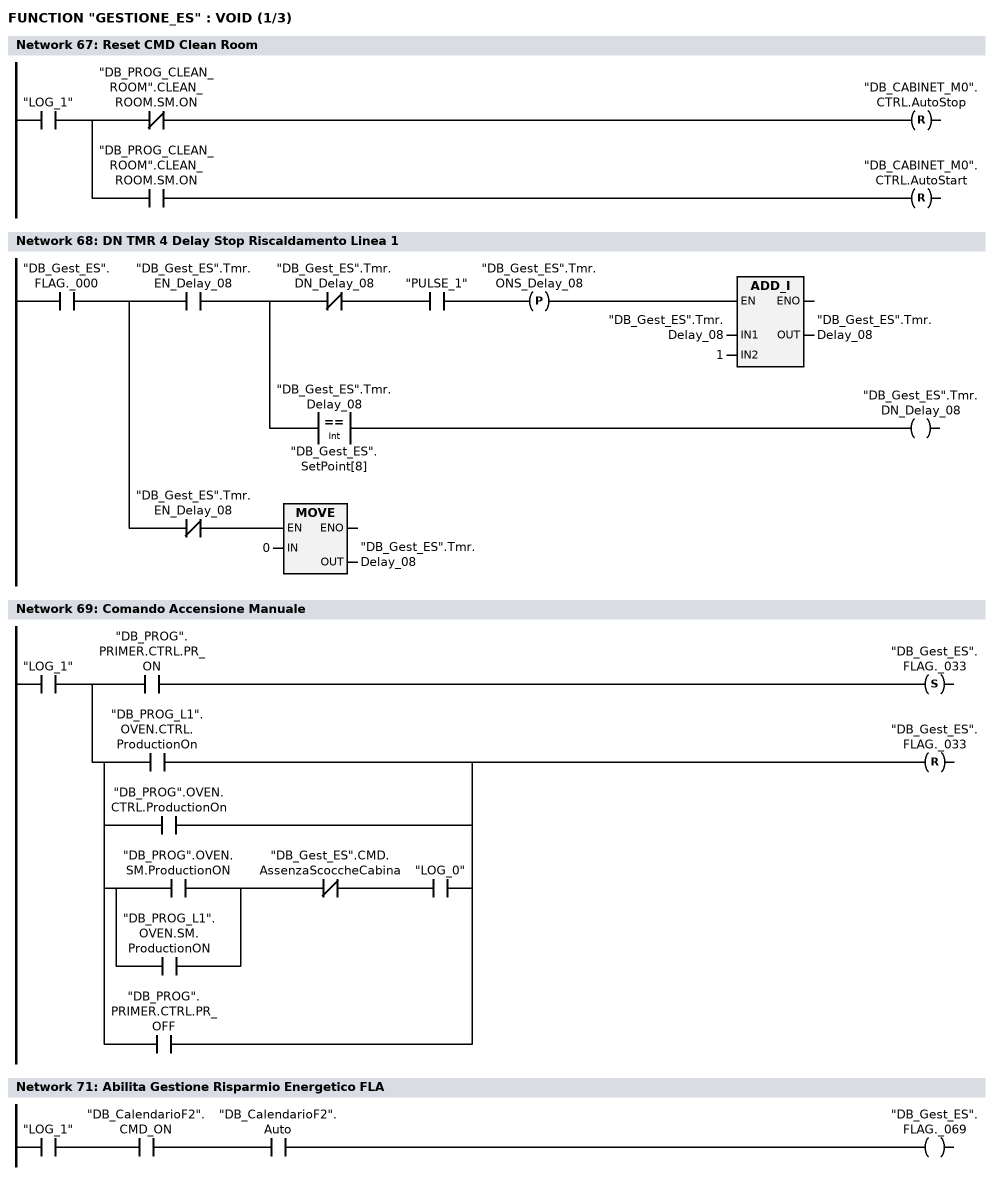
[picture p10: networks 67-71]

      U     "LOG_1";
      =     L     22.0;
      U     L     22.0;
      UN    "DB_PROG_CLEAN_ROOM".CLEAN_ROOM.SM.ON;
      R     "DB_CABINET_M0".CTRL.AutoStop;
      U     L     22.0;
      U     "DB_PROG_CLEAN_ROOM".CLEAN_ROOM.SM.ON;
      R     "DB_CABINET_M0".CTRL.AutoStart;
NETWORK
TITLE =DN TMR 4 Delay Stop Riscaldamento Linea 1

      U     "DB_Gest_ES".FLAG._000;
      =     L     22.0;
      U     L     22.0;
      U     "DB_Gest_ES".Tmr.EN_Delay_08;
      =     L     22.1;
      U     L     22.1;
      UN    "DB_Gest_ES".Tmr.DN_Delay_08;
      U     "PULSE_1";
      FP    "DB_Gest_ES".Tmr.ONS_Delay_08;
      SPBNB _018;
      L     "DB_Gest_ES".Tmr.Delay_08;
      L     1;
      +I    ;
      T     "DB_Gest_ES".Tmr.Delay_08;
_018: NOP   0;
      U     L     22.1;
      U(    ;
      L     "DB_Gest_ES".Tmr.Delay_08;
      L     "DB_Gest_ES".SetPoint[8];
      ==I   ;
      )     ;
      =     "DB_Gest_ES".Tmr.DN_Delay_08;
      U     L     22.0;
      UN    "DB_Gest_ES".Tmr.EN_Delay_08;
      SPBNB _019;
      L     0;
      T     "DB_Gest_ES".Tmr.Delay_08;
_019: NOP   0;
NETWORK
TITLE =Comando Accensione Manuale

      U     "LOG_1";
      =     L     22.0;
      U     L     22.0;
      U     "DB_PROG".PRIMER.CTRL.PR_ON;
      S     "DB_Gest_ES".FLAG._033;
      U     L     22.0;
      U(    ;
      O     "DB_PROG_L1".OVEN.CTRL.ProductionOn;
      O     "DB_PROG".OVEN.CTRL.ProductionOn;
      O     ;
      U(    ;
      O     "DB_PROG".OVEN.SM.ProductionON;
      O     "DB_PROG_L1".OVEN.SM.ProductionON;
      )     ;
      UN    "DB_Gest_ES".CMD.AssenzaScoccheCabina;
      U     "LOG_0";
      O     "DB_PROG".PRIMER.CTRL.PR_OFF;
      )     ;
      R     "DB_Gest_ES".FLAG._033;
NETWORK
TITLE =########################

NETWORK
TITLE =Abilita Gestione Risparmio Energetico FLA

      U     "LOG_1";
      U     "DB_CalendarioF2".CMD_ON;
      U     "DB_CalendarioF2".Auto;
      =     "DB_Gest_ES".FLAG._069;
NETWORK
TITLE =Set Point
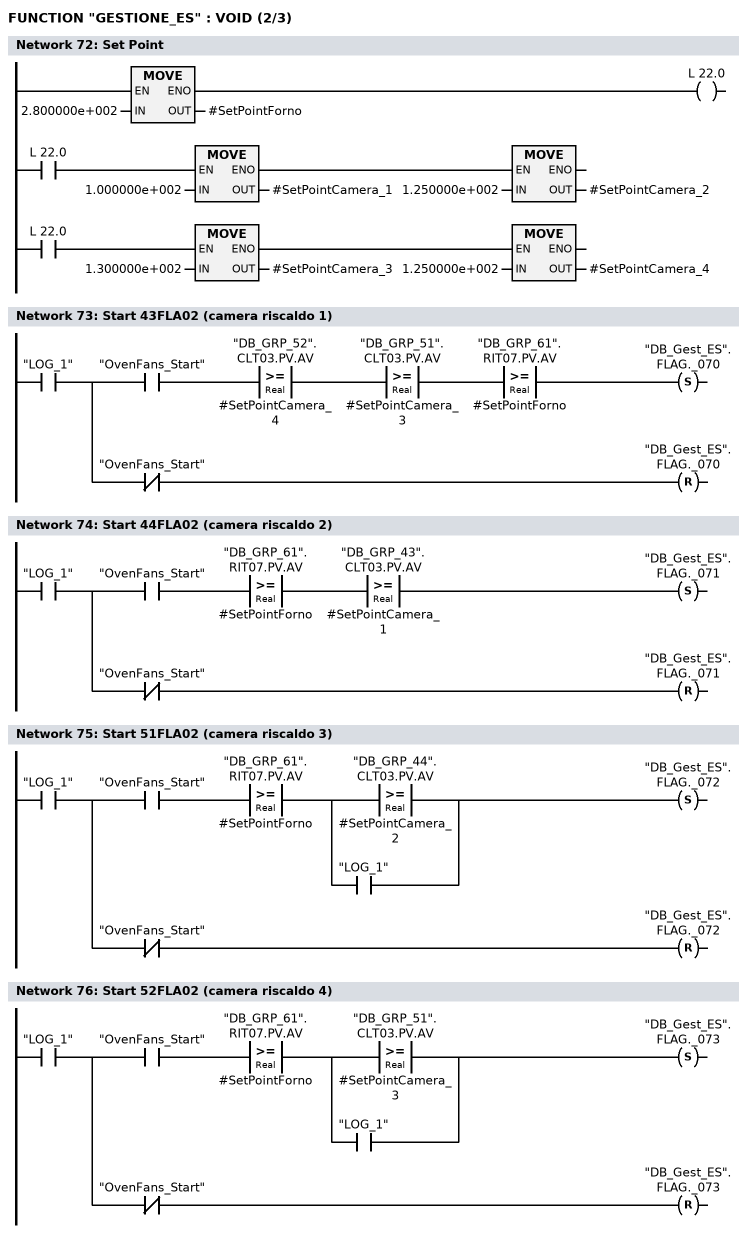
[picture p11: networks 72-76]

      L     2.800000e+002;
      T     #SetPointForno;
      SET   ;
      SAVE  ;
      CLR   ;
      U     BIE;
      =     L     22.0;
      U(    ;
      U     L     22.0;
      SPBNB _01a;
      L     1.000000e+002;
      T     #SetPointCamera_1;
      SET   ;
      SAVE  ;
      CLR   ;
_01a: U     BIE;
      )     ;
      SPBNB _01b;
      L     1.250000e+002;
      T     #SetPointCamera_2;
_01b: NOP   0;
      U(    ;
      U     L     22.0;
      SPBNB _01c;
      L     1.300000e+002;
      T     #SetPointCamera_3;
      SET   ;
      SAVE  ;
      CLR   ;
_01c: U     BIE;
      )     ;
      SPBNB _01d;
      L     1.250000e+002;
      T     #SetPointCamera_4;
_01d: NOP   0;
NETWORK
TITLE =Start 43FLA02 (camera riscaldo 1)

      U     "LOG_1";
      =     L     22.0;
      U     L     22.0;
      U     "OvenFans_Start";
      U(    ;
      L     "DB_GRP_52".CLT03.PV.AV;
      L     #SetPointCamera_4;
      >=R   ;
      )     ;
      U(    ;
      L     "DB_GRP_51".CLT03.PV.AV;
      L     #SetPointCamera_3;
      >=R   ;
      )     ;
      U(    ;
      L     "DB_GRP_61".RIT07.PV.AV;
      L     #SetPointForno;
      >=R   ;
      )     ;
      S     "DB_Gest_ES".FLAG._070;
      U     L     22.0;
      UN    "OvenFans_Start";
      R     "DB_Gest_ES".FLAG._070;
NETWORK
TITLE =Start 44FLA02 (camera riscaldo 2)

      U     "LOG_1";
      =     L     22.0;
      U     L     22.0;
      U     "OvenFans_Start";
      U(    ;
      L     "DB_GRP_61".RIT07.PV.AV;
      L     #SetPointForno;
      >=R   ;
      )     ;
      U(    ;
      L     "DB_GRP_43".CLT03.PV.AV;
      L     #SetPointCamera_1;
      >=R   ;
      )     ;
      S     "DB_Gest_ES".FLAG._071;
      U     L     22.0;
      UN    "OvenFans_Start";
      R     "DB_Gest_ES".FLAG._071;
NETWORK
TITLE =Start 51FLA02 (camera riscaldo 3)

      U     "LOG_1";
      =     L     22.0;
      U     L     22.0;
      U     "OvenFans_Start";
      U(    ;
      L     "DB_GRP_61".RIT07.PV.AV;
      L     #SetPointForno;
      >=R   ;
      )     ;
      U(    ;
      O(    ;
      L     "DB_GRP_44".CLT03.PV.AV;
      L     #SetPointCamera_2;
      >=R   ;
      )     ;
      O     "LOG_1";
      )     ;
      S     "DB_Gest_ES".FLAG._072;
      U     L     22.0;
      UN    "OvenFans_Start";
      R     "DB_Gest_ES".FLAG._072;
NETWORK
TITLE =Start 52FLA02 (camera riscaldo 4)

      U     "LOG_1";
      =     L     22.0;
      U     L     22.0;
      U     "OvenFans_Start";
      U(    ;
      L     "DB_GRP_61".RIT07.PV.AV;
      L     #SetPointForno;
      >=R   ;
      )     ;
      U(    ;
      O(    ;
      L     "DB_GRP_51".CLT03.PV.AV;
      L     #SetPointCamera_3;
      >=R   ;
      )     ;
      O     "LOG_1";
      )     ;
      S     "DB_Gest_ES".FLAG._073;
      U     L     22.0;
      UN    "OvenFans_Start";
      R     "DB_Gest_ES".FLAG._073;
NETWORK
TITLE =***** Gestione Cabina ******

NETWORK
TITLE =Modalita 1 Estate
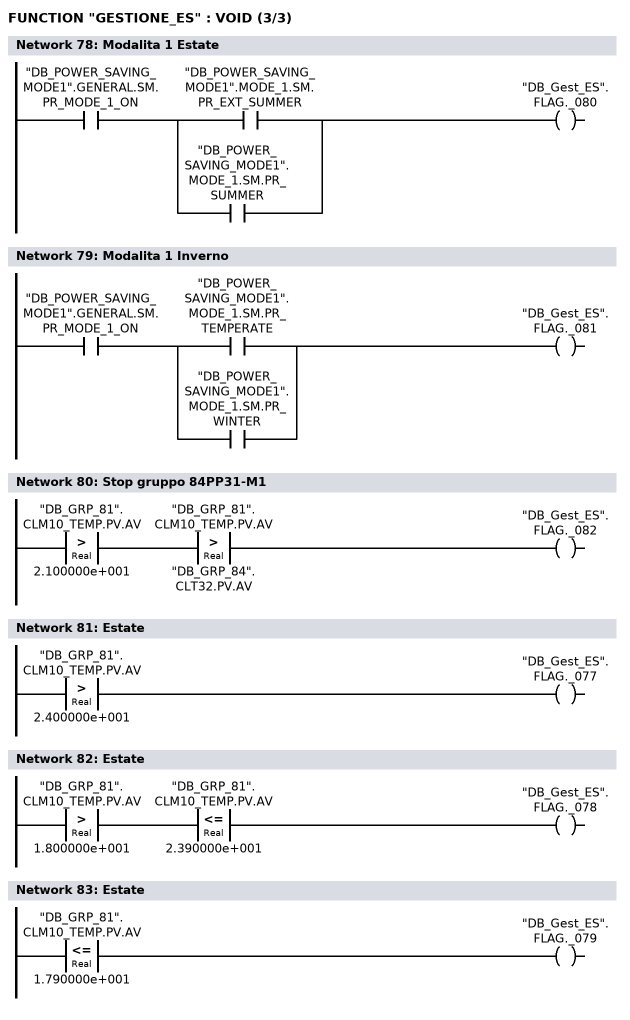
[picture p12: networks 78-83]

      U     "DB_POWER_SAVING_MODE1".GENERAL.SM.PR_MODE_1_ON;
      U(    ;
      O     "DB_POWER_SAVING_MODE1".MODE_1.SM.PR_EXT_SUMMER;
      O     "DB_POWER_SAVING_MODE1".MODE_1.SM.PR_SUMMER;
      )     ;
      =     "DB_Gest_ES".FLAG._080;
NETWORK
TITLE =Modalita 1 Inverno

      U     "DB_POWER_SAVING_MODE1".GENERAL.SM.PR_MODE_1_ON;
      U(    ;
      O     "DB_POWER_SAVING_MODE1".MODE_1.SM.PR_TEMPERATE;
      O     "DB_POWER_SAVING_MODE1".MODE_1.SM.PR_WINTER;
      )     ;
      =     "DB_Gest_ES".FLAG._081;
NETWORK
TITLE =Stop gruppo 84PP31-M1

      U(    ;
      L     "DB_GRP_81".CLM10_TEMP.PV.AV;
      L     2.100000e+001;
      >R    ;
      )     ;
      U(    ;
      L     "DB_GRP_81".CLM10_TEMP.PV.AV;
      L     "DB_GRP_84".CLT32.PV.AV;
      >R    ;
      )     ;
      =     "DB_Gest_ES".FLAG._082;
NETWORK
TITLE =Estate

      L     "DB_GRP_81".CLM10_TEMP.PV.AV;
      L     2.400000e+001;
      >R    ;
      =     "DB_Gest_ES".FLAG._077;
NETWORK
TITLE =Estate

      U(    ;
      L     "DB_GRP_81".CLM10_TEMP.PV.AV;
      L     1.800000e+001;
      >R    ;
      )     ;
      U(    ;
      L     "DB_GRP_81".CLM10_TEMP.PV.AV;
      L     2.390000e+001;
      <=R   ;
      )     ;
      =     "DB_Gest_ES".FLAG._078;
NETWORK
TITLE =Estate

      L     "DB_GRP_81".CLM10_TEMP.PV.AV;
      L     1.790000e+001;
      <=R   ;
      =     "DB_Gest_ES".FLAG._079;
END_FUNCTION

